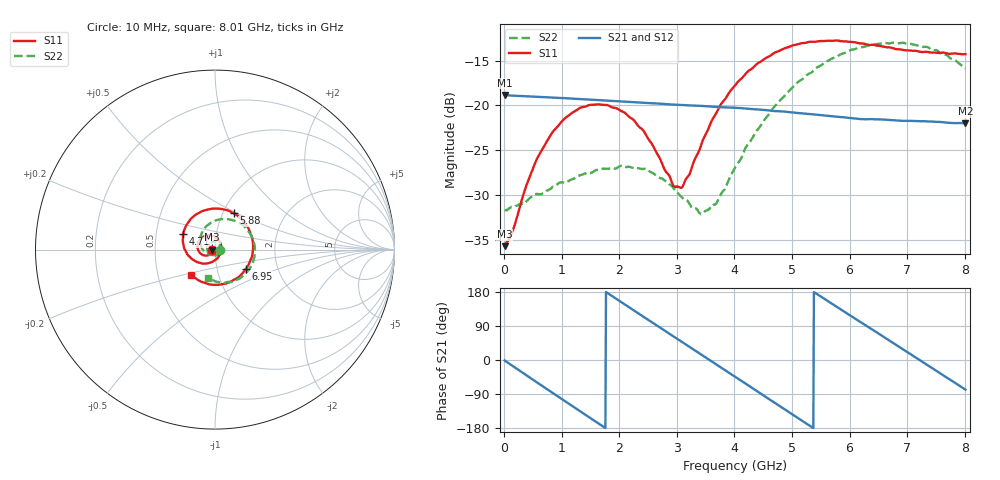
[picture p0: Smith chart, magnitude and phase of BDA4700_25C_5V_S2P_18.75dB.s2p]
!Agilent Technologies,E5071B,MY42404982,A.09.10
!Date: Mon Oct 20 13:35:43 2025
!Data & Calibration Information:
!Freq	S11:SOLT2(ON)	S21:SOLT2(ON)	S12:SOLT2(ON)	S22:SOLT2(ON)
# Hz S RI R 50
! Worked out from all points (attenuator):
!   801 points, 10 MHz to 8.01 GHz, reference 50 ohm
!   highest |S21| = -18.84 dB at 10 MHz (marker M1); lowest = -22.0 dB at 8.01 GHz (marker M2)
!   lowest |S11| = -35.7 dB at 10 MHz (marker M3), VSWR 1.03, Z = 48.4 - j0.114 ohm
!   |S11| at or under -10 dB: start of sweep to end of sweep
!   |S22| runs from -32.1 to -13.0 dB; largest |S21 - S12| = 0.00089
!   S11 on the Smith chart (normalised r, x): 10 MHz: 0.97, -0.00; 4.71 GHz: 0.69, +0.12; 5.88 GHz: 1.12, +0.48; 6.95 GHz: 1.38, -0.30; 8.01 GHz: 0.74, -0.21
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1e7  -0.0164 -0.00118  0.1143 -0.00245  0.1142 -0.00257  0.0261 -0.00085
1.5e8  -0.0177 -0.00967  0.1091 -0.0309  0.1091 -0.0309  0.0263 -0.0072
3.9e8  -0.0264 -0.0246  0.0855 -0.073  0.0855 -0.0731  0.021 -0.0205
6.3e8  -0.0433 -0.0332  0.0471 -0.1011  0.0471 -0.1011  0.0106 -0.0303
1.01e9  -0.0786 -0.0236  -0.026 -0.1068  -0.026 -0.1068  -0.0162 -0.0337
1.35e9  -0.0974 0.00832  -0.0808 -0.0723  -0.0808 -0.0723  -0.0374 -0.0171
2.08e9  -0.0476 0.0784  -0.0893 0.0553  -0.0893 0.0553  -0.0282 0.0359
2.42e9  -0.00146 0.0723  -0.0424 0.0944  -0.0424 0.0944  -0.00185 0.0442
2.68e9  0.0254 0.0458  0.00299 0.1023  0.00298 0.1023  0.0162 0.0364
2.94e9  0.0348 0.0082  0.0467 0.0896  0.0468 0.0896  0.0275 0.0213
3.09e9  0.0314 -0.0155  0.0681 0.0742  0.0677 0.0743  0.0294 0.00903
3.46e9  -0.00723 -0.0646  0.0975 0.0185  0.0975 0.0185  0.0166 -0.0192
3.69e9  -0.0487 -0.0773  0.096 -0.0205  0.096 -0.0208  -0.00183 -0.0285
4.01e9  -0.1127 -0.0628  0.0698 -0.0674  0.0698 -0.0673  -0.0358 -0.0271
4.71e9  -0.178 0.0858  -0.0378 -0.085  -0.0377 -0.0852  -0.0828 0.0557
5.35e9  -0.06 0.2181  -0.0892 -0.00363  -0.0893 -0.00391  -0.0135 0.153
5.88e9  0.1033 0.2027  -0.0555 0.0658  -0.0555 0.0657  0.109 0.1609
6.25e9  0.1868 0.1176  -0.00678 0.0835  -0.00589 0.0836  0.186 0.1024
6.68e9  0.2093 -0.0233  0.0507 0.0657  0.0509 0.0657  0.2215 -0.00753
6.95e9  0.1735 -0.1053  0.0736 0.0364  0.0738 0.0359  0.2074 -0.0808
7.48e9  0.0251 -0.1952  0.0729 -0.0356  0.073 -0.0357  0.0976 -0.1783
8.01e9  -0.1326 -0.1399  0.0163 -0.078  0.0164 -0.0781  -0.0371 -0.156
